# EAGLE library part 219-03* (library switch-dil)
Surface Mount DIP Switch Series 219 SMT CTS Electronic Components Sourc: www.ctscorp.com
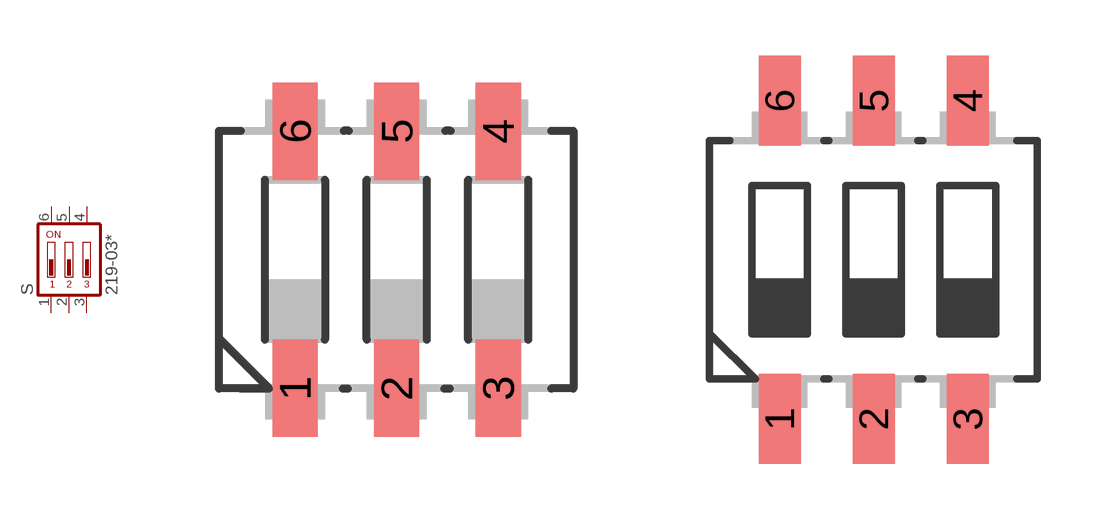
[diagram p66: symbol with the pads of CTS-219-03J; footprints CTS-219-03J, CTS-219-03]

Designator prefix S

## 219-03J (OC_FARNELL: unknown; OC_NEWARK: unknown)  [CTS-219-03J]
1  1  pas
2  2  pas
3  3  pas
4  4  pas
5  5  pas
6  6  pas

## 219-03 (OC_FARNELL: unknown; OC_NEWARK: unknown)  [CTS-219-03]
Pads as for CTS-219-03J

## Footprint CTS-219-03J (pad centres in mm)
Surface Mount DIP Switch Series 219 SMT "J" Bend CTS Electronic Components Sourc: www.ctscorp.com
smd 1.13 x 2.44: 1 -2.54,-3.215; 2 0,-3.215; 3 2.54,-3.215; 4 2.54,3.215; 5 0,3.215; 6 -2.54,3.215

## Footprint CTS-219-03 (pad centres in mm)
Surface Mount DIP Switch Series 219 SMT CTS Electronic Components Sourc: www.ctscorp.com
smd 1.13 x 2.44: 1 -2.54,-4.3; 2 0,-4.3; 3 2.54,-4.3; 4 2.54,4.3; 5 0,4.3; 6 -2.54,4.3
